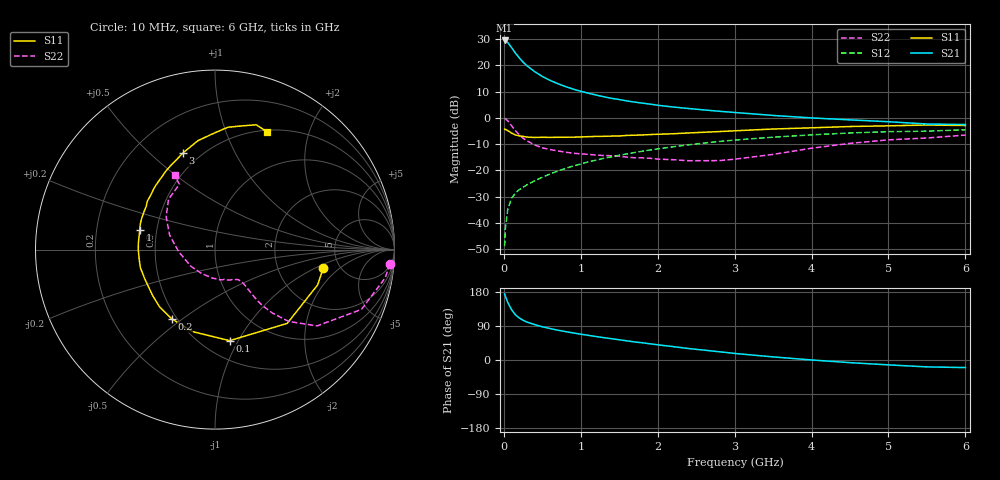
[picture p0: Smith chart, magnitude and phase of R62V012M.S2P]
! SIEMENS Small Signal Semiconductors
! BFR193
! Si NPN RF Bipolar Junction Transistor in SOT23
! VCE = 2 V  IC = 12 mA
! Common Emitter S-Parameters:  May  1996
# GHz  S  MA  R  50
!  f  S11  S21  S12  S22
! GHz  MAG  ANG  MAG  ANG  MAG  ANG  MAG  ANG
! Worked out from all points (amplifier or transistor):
!   36 points, 10 MHz to 6 GHz, reference 50 ohm
!   highest |S21| = 29.5 dB at 10 MHz (marker M1)
!   |S21| within 3 dB of that: start of sweep to 107.1 MHz
!   unconditionally stable (mu >= 1): 674.6 MHz to 2.004 GHz
!   at 250 MHz: K = 0.70, MSG = 23.9 dB, |S12| = -26.4 dB
!   at 1.4 GHz: K = 1.04, MAG = 10.0 dB, |S12| = -14.8 dB
!   at 6 GHz: K = 0.95, MSG = 1.0 dB, |S12| = -4.5 dB
!   S11 on the Smith chart (normalised r, x): 10 MHz: 3.71, -1.23; 100 MHz: 0.67, -0.92; 200 MHz: 0.47, -0.46; 1 GHz: 0.40, +0.11; 3 GHz: 0.40, +0.64; 6 GHz: 0.52, +1.41
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0.01  0.6116 -9.8  29.89 174.2  0.0036 86.4  0.977 -4.7
0.02  0.6049 -18.9  29.59 168.2  0.0078 80.6  0.9614 -9.4
0.05  0.5752 -45.6  27.5 152.4  0.0178 73.5  0.8816 -22.2
0.1  0.514 -80.8  21.9 132.8  0.0294 62.2  0.71 -36.8
0.15  0.4738 -105.4  17.23 119.4  0.0369 57.4  0.5726 -44.3
0.2  0.4547 -122.1  13.98 111.0  0.0429 56.7  0.4757 -47.9
0.25  0.4445 -133.9  11.56 104.8  0.0476 56.9  0.4105 -49.7
0.3  0.4316 -143.6  9.861 100.1  0.053 58.2  0.366 -50.3
0.4  0.424 -157.3  7.629 93.4  0.0634 60.2  0.305 -50.3
0.5  0.4278 -166.3  6.155 87.7  0.074 62.1  0.269 -50.0
0.6  0.4258 -173.5  5.188 83.1  0.0854 63.1  0.2494 -50.0
0.7  0.4274 -179.9  4.5 78.7  0.0969 63.6  0.2349 -50.5
0.8  0.4285 175.3  3.953 75.0  0.1088 63.9  0.2226 -51.3
1  0.4334 165.3  3.214 68.1  0.1327 63.9  0.2068 -53.7
1.1  0.4396 161.3  2.951 65.0  0.1451 63.5  0.2017 -56.0
1.6  0.4639 144.3  2.103 50.5  0.2063 59.6  0.1794 -69.6
2.2  0.4989 127.3  1.613 35.3  0.2818 52.9  0.1599 -94.6
3  0.568 108.2  1.27 17.3  0.3783 41.6  0.1634 -145.3
3.5  0.6144 98.9  1.114 8.2  0.4294 33.8  0.2015 -176.1
4.5  0.6854 84.0  0.917 -7.0  0.5165 19.1  0.3276 146.2
5.5  0.7323 71.7  0.765 -18.2  0.5583 4.1  0.4142 118.6
6  0.7169 66.0  0.747 -20.0  0.5949 -0.4  0.471 118.5
